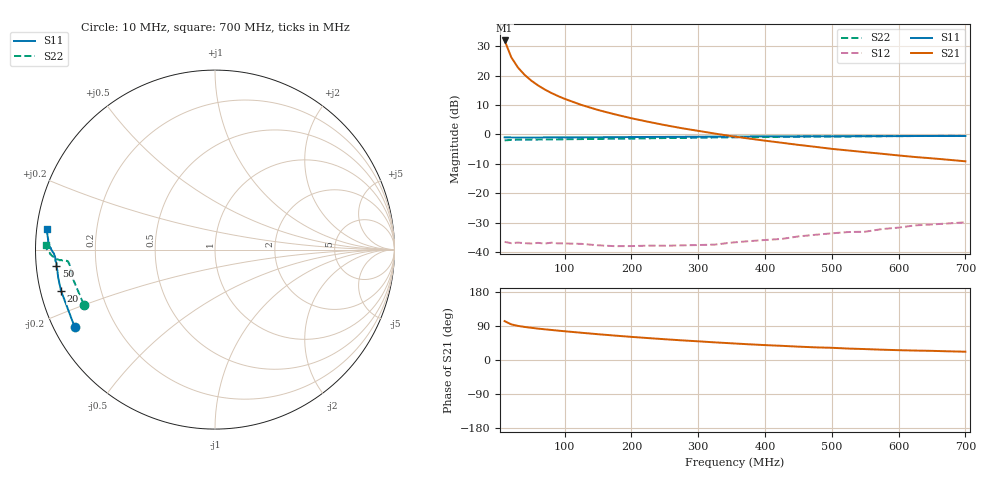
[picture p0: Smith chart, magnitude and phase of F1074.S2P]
! Date: Mon Aug 07 16:58:30 1995
# MHZ  S  MA  R  50.0000
!  POLYFET RF DEVICES
!  F1074 (Each Side)
!  S PARAMETERS
!  VDS=28V, IDQ=800mA
!FREQ  S11MAG S11ANG S21MAG S21ANG S12MAG S12ANG S22MAG S22ANG
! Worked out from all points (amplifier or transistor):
!   34 points, 10 MHz to 700 MHz, reference 50 ohm
!   highest |S21| = 32.0 dB at 10 MHz (marker M1)
!   |S21| within 3 dB of that: start of sweep to 15.24 MHz
!   unconditionally stable (mu >= 1): 244.3 MHz to 449.8 MHz; 494.3 MHz to 503.2 MHz
!   at 60 MHz: K = 0.26, MSG = 26.8 dB, |S12| = -36.9 dB
!   at 300 MHz: K = 1.15, MAG = 17.1 dB, |S12| = -37.6 dB
!   at 700 MHz: K = 0.73, MSG = 10.4 dB, |S12| = -29.9 dB
!   S11 on the Smith chart (normalised r, x): 10 MHz: 0.06, -0.26; 20 MHz: 0.06, -0.13; 50 MHz: 0.06, -0.05; 700 MHz: 0.03, +0.06
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10  0.8932 -151.1  39.58 102.6  0.01491 15.1  0.7931 -157.3
20  0.888 -165.0  20.47 93.9  0.01417 7.2  0.8071 -168.1
30  0.8874 -169.9  13.7 90.0  0.01451 6.9  0.8119 -171.6
40  0.8859 -172.4  10.28 87.3  0.01418 5.8  0.8126 -173.4
50  0.8882 -174.1  8.206 85.0  0.01398 5.7  0.816 -174.4
60  0.8857 -175.0  6.818 82.9  0.01436 5.0  0.8193 -174.9
70  0.8889 -175.6  5.818 81.0  0.01395 6.3  0.8201 -175.1
80  0.8914 -176.0  5.068 79.3  0.01445 5.2  0.8206 -175.4
90  0.8908 -176.7  4.488 77.5  0.01406 6.5  0.8246 -175.5
100  0.8915 -177.0  4.023 75.9  0.01404 5.8  0.8268 -175.6
125  0.8924 -177.6  3.175 71.9  0.0138 10.4  0.8333 -175.7
150  0.8955 -178.1  2.603 68.0  0.01305 11.2  0.8386 -175.9
175  0.898 -178.7  2.198 64.4  0.01261 14.6  0.8471 -175.9
200  0.9029 -179.1  1.883 61.0  0.01266 21.9  0.85 -175.9
225  0.9061 -179.3  1.641 57.8  0.01287 24.4  0.8591 -176.1
250  0.909 -179.7  1.441 54.8  0.01284 28.1  0.8676 -176.1
300  0.9146 179.5  1.15 49.3  0.01318 37.4  0.879 -176.5
375  0.9233 178.5  0.854 41.5  0.01532 51.9  0.8978 -177.2
475  0.9315 176.7  0.6161 33.4  0.01968 61.8  0.9186 -178.4
550  0.9344 175.6  0.4995 28.8  0.02221 66.9  0.9291 -179.5
600  0.9366 174.9  0.4393 25.9  0.02609 70.5  0.936 179.9
700  0.9432 173.0  0.3494 21.9  0.03211 70.5  0.9418 178.6
